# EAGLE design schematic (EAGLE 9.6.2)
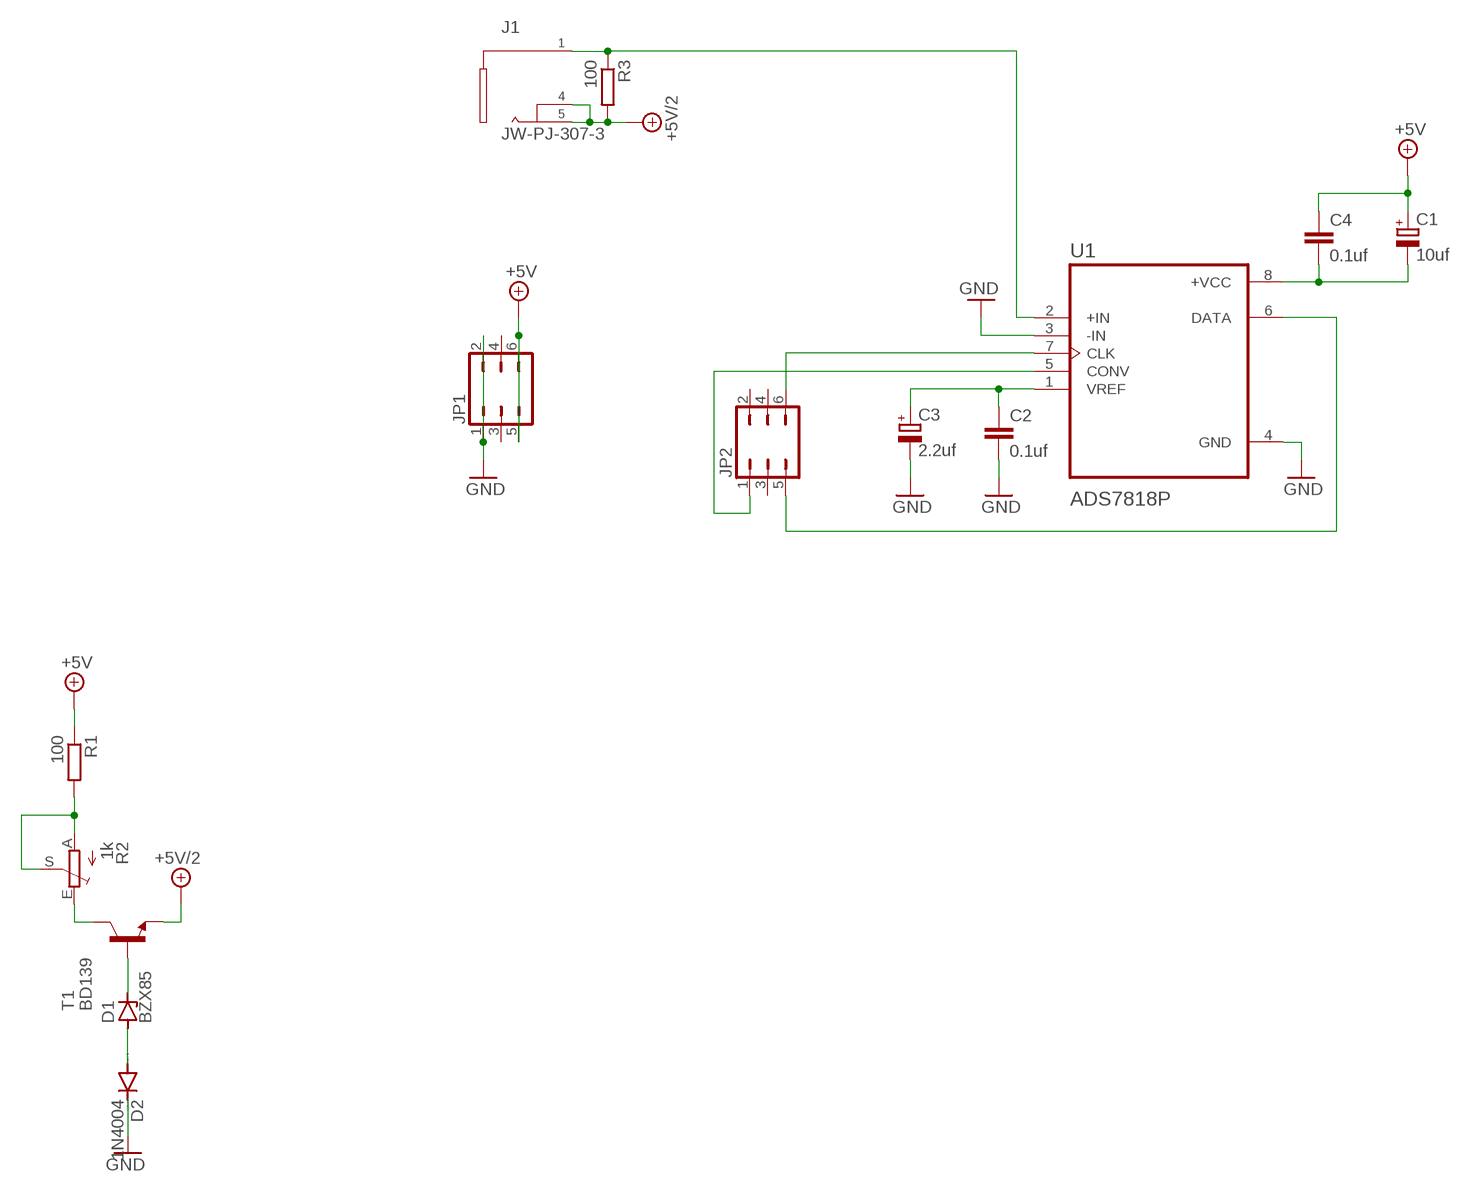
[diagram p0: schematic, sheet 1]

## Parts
C1  10uf  CPOL-EUE3.5-8  [E3,5-8]
C2  0.1uf  C-EU050-030X075  [C050-030X075]
C3  2.2uf  CPOL-EUE2.5-6  [E2,5-6]
C4  0.1uf  C-EU050-030X075  [C050-030X075]
D1  BZX85  [DO41Z10]
D2  1N4004  [DO41-10]
J1  JW-PJ-307-3  [JW-PJ-307-X]
JP1  JP3Q  [JP3Q]
JP2  JP3Q  [JP3Q]
R1  100  R-EU_0207/10  [0207/10]
R2  1k  TRIM_EU-CA9V  [CA9V]
R3  100  R-EU_0207/10  [0207/10]
T1  BD139  [TO126]
U1  ADS7818P  [DIP794W45P254L959H508Q8]

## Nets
+5V: C1.+ C4.1 JP1.5 JP1.6 R1.1
+5V/2: J1.P$4 J1.P$5 R3.2 T1.1(E)
GND: C2.2 C3.- D2.C JP1.1 JP1.2 U1.3(-IN) U1.4(GND)
N$1: R1.2 R2.A R2.S
N$2: D1.A D2.A
N$3: D1.C T1.3(B)
N$4: R2.E T1.2(C)
N$5: JP2.6 U1.7(CLK)
N$6: J1.P$1 R3.1 U1.2(+IN)
N$7: JP2.1 U1.5(CONV)
N$8: C2.1 C3.+ U1.1(VREF)
N$9: JP2.5 U1.6(DATA)
N$10: C1.- C4.2 U1.8(+VCC)
Unconnected: JP1.3 JP1.4 JP2.2 JP2.3 JP2.4

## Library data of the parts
C1 C3 = rcl:CPOL-EU: POLARIZED CAPACITOR, European symbol; SPICEPREFIX: C
C2 C4 = rcl:C-EU: CAPACITOR, European symbol; SPICEPREFIX: C
D1 = diode:BZX85: Z DIODE
D2 = diode:1N4004: DIODE
J1 = audioconn:JW-PJ-307-3
JP1 JP2 = jumper:JP3Q: JUMPER
R1 R3 = rcl:R-EU_: RESISTOR, European symbol; SPICEPREFIX: R
R2 = pot:TRIM_EU-: POTENTIOMETER
T1 = transistor:BD139: NPN TRANSISTOR
U1 = ADS7818P:ADS7818P: Check prices; AVAILABILITY: Warning; DESCRIPTION: 12-Bit High Speed Low Power Sampling Analog-to-Digital Converter; MF: Texas Instruments; MP: ADS7818P; PACKAGE: PDIP-8 Texas; PRICE: None; PURCHASE-URL: https://pricing.snapeda.com/search/part/ADS7818P/?ref=eda

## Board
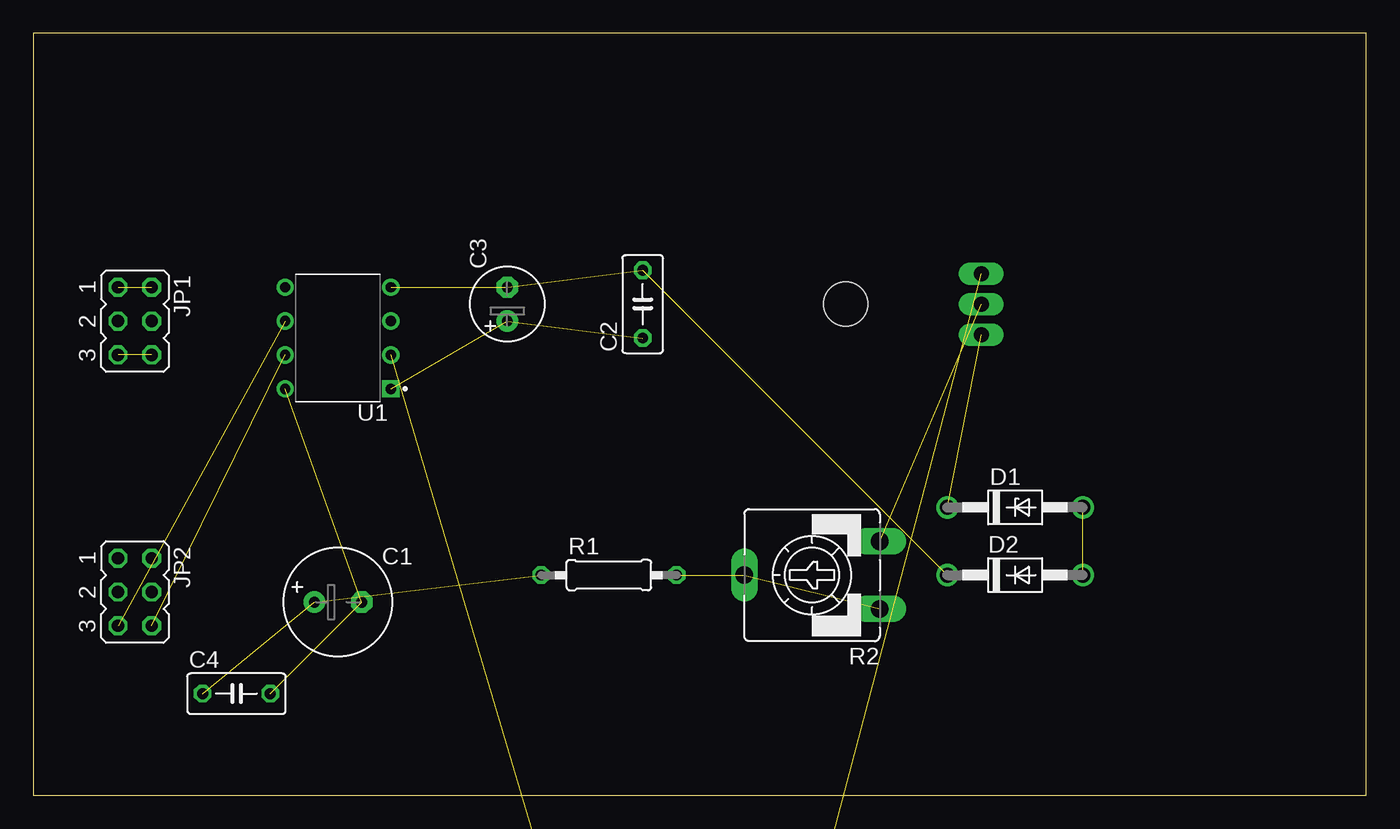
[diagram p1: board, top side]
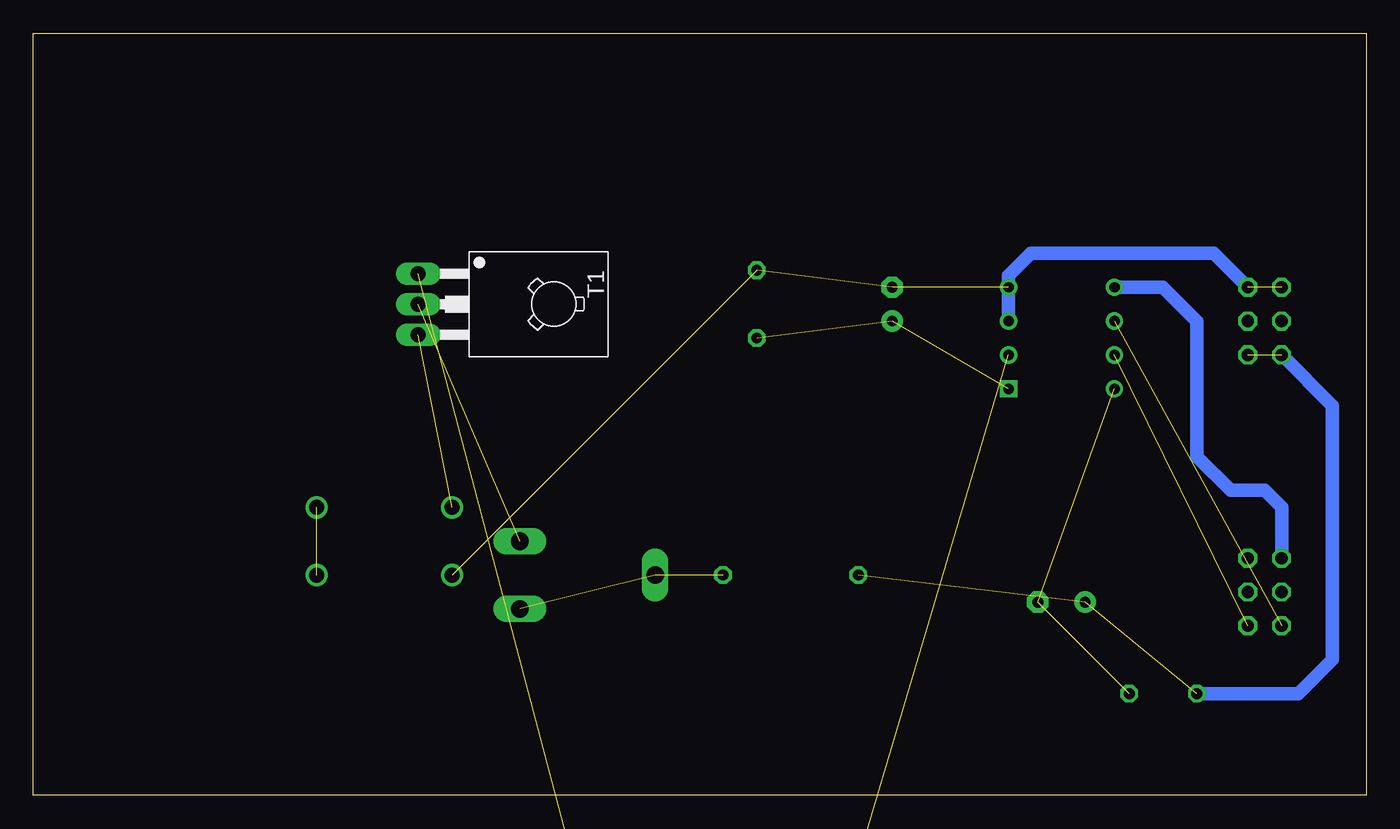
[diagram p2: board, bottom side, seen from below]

Size 100 x 57.14 mm. Coordinates in mm from the lower left corner, seen from the top.
Outline: 0,0 100,0 100,57.14 0,57.14 0,0
Copper layers (1*16): Top 0.035mm / dielectric 1.5mm / Bottom 0.035mm
Design rules "default": minimum track width 6mil, minimum drill 0.35mm, track to track 6mil, track to pad 6mil, pad to pad 6mil, via to via 6mil, smd to smd 6mil, copper to edge 40mil, drill to drill 6mil, minimum pad ring 10mil, minimum via ring 8mil, stop-mask expansion 4mil, vias tented up to drill 0mil, thermal gap 10mil

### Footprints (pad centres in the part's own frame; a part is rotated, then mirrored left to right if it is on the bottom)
E3,5-8 = drill 0.813 pad 1.6: + -1.778,0 | drill 0.813 pad 1.6 octagon: - 1.778,0
C050-030X075 = drill 0.813 octagon: 1 -2.54,0; 2 2.54,0
E2,5-6 = drill 0.813 pad 1.6: + -1.27,0 | drill 0.813 pad 1.6 octagon: - 1.27,0
DO41Z10 = drill 1.118: A 5.08,0; C -5.08,0
DO41-10 = drill 1.118: A 5.08,0; C -5.08,0
JW-PJ-307-X = drill 0.7 pad 1.422 long: P$1 3,2.5; P$2 3,5; P$3 3,-2.5; P$4 3,-5; P$5 -2,0.5 | hole 1.2: -4.5,5; -2,5; 3,0; -4.5,-5; -2,-5
JP3Q = drill 0.914 octagon: 1 -2.54,-1.27; 2 -2.54,1.27; 3 0,-1.27; 4 0,1.27; 5 2.54,-1.27; 6 2.54,1.27
0207/10 = drill 0.813 octagon: 1 -5.08,0; 2 5.08,0
CA9V = drill 1.321 long: A -2.54,-5.08; E 2.54,-5.08; S 0,5.08
TO126 = drill 1.118 long: 1 -2.286,-5.08; 2 0,-5.08; 3 2.286,-5.08 | hole 3.302: 0,5.08
DIP794W45P254L959H508Q8 = drill 0.78 pad 1.13 square: 1 -3.97,3.81 | drill 0.78 pad 1.13: 2 -3.97,1.27; 3 -3.97,-1.27; 4 -3.97,-3.81; 5 3.97,-3.81; 6 3.97,-1.27; 7 3.97,1.27; 8 3.97,3.81

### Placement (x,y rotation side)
C1  22.86,14.48 0 top
C2  45.72,36.83 90 top
C3  35.56,36.83 90 top
C4  15.24,7.62 0 top
D1  73.66,21.59 0 top
D2  73.66,16.51 0 top
J1  not placed on the board
JP1  7.62,35.56 270 top
JP2  7.62,15.24 270 top
R1  43.18,16.51 0 top
R2  58.42,16.51 90 top
R3  not placed on the board
T1  66.04,36.83 270 bottom
U1  22.86,34.29 180 top

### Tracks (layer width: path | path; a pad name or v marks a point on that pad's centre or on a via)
+5V  (3 unrouted)
  Bottom 1: JP1.5 2.54,29.21 2.54,10.16 5.08,7.62 C4.1
+5V/2  (3 unrouted)
GND  (4 unrouted)
  Bottom 1: JP1.2 11.43,40.64 25.15,40.64 26.83,38.96 U1.4 U1.3
N$1  (2 unrouted)
N$2  (1 unrouted)
N$3  (1 unrouted)
N$4  (1 unrouted)
N$5  (1 unrouted)
N$6  (2 unrouted)
N$7
  Bottom 1: U1.5 15.24,38.1 12.7,35.56 12.7,25.4 10.16,22.86 7.62,22.86 6.35,21.59 JP2.1
N$8  (2 unrouted)
N$9  (1 unrouted)
N$10  (2 unrouted)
